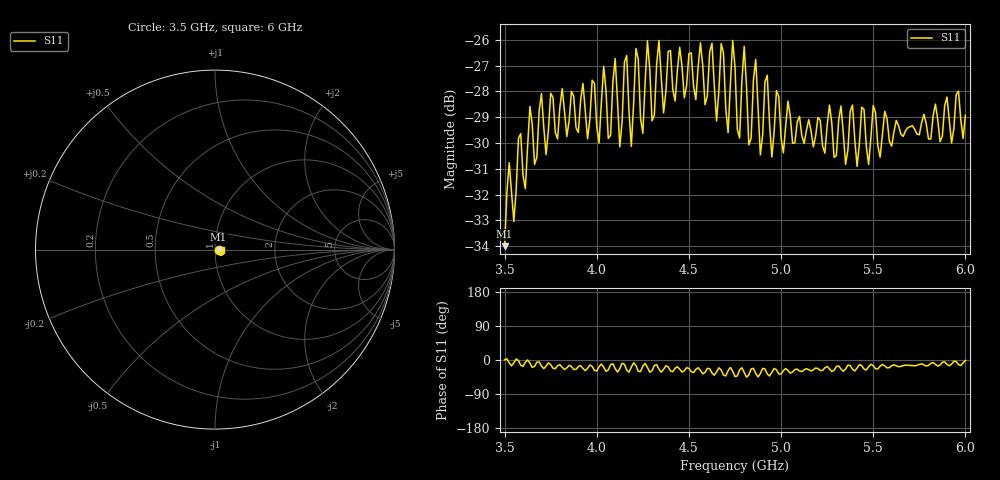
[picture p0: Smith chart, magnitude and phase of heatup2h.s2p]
!  31/07/2025  12:56:16
! Ref Plane: 0.000 mm
# MHZ S MA R  50
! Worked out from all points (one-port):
!   201 points, 3.5 GHz to 6 GHz, reference 50 ohm
!   lowest |S11| = -34.0 dB at 3.5 GHz (marker M1), VSWR 1.04, Z = 52 + j0.017 ohm
!   |S11| at or under -10 dB: start of sweep to end of sweep
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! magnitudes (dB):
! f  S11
! 3.5 GHz  -34.0
! 3.525 GHz  -30.8
! 3.55 GHz  -33.0
! 3.638 GHz  -28.6
! 3.812 GHz  -27.9
! 4.013 GHz  -30.0
! 4.037 GHz  -27.0
! 4.062 GHz  -29.8
! 4.1 GHz  -26.7
! 4.125 GHz  -30.2
! 4.162 GHz  -26.6
! 4.188 GHz  -30.1
! 4.213 GHz  -26.3
! 4.25 GHz  -29.6
! 4.275 GHz  -26.0
! 4.3 GHz  -29.1
! 4.338 GHz  -26.0
! 4.362 GHz  -28.8
! 4.438 GHz  -27.2
! 4.625 GHz  -26.1
! 4.65 GHz  -29.1
! 4.675 GHz  -26.1
! 4.713 GHz  -29.6
! 4.75 GHz  -27.1
! 5.062 GHz  -30.0
! 5.375 GHz  -28.8
! 5.688 GHz  -29.4
! 6 GHz  -28.9
